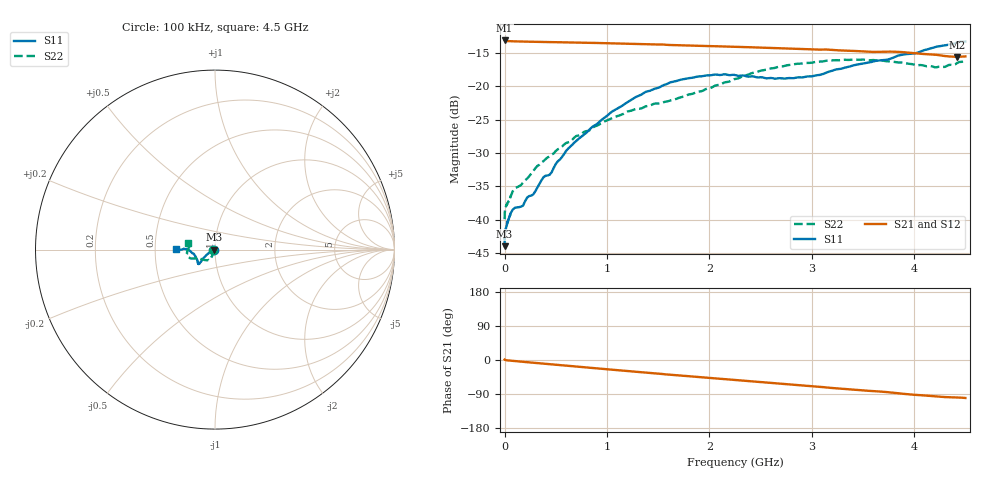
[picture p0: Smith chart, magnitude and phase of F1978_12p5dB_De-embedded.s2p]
! Integrated Device Technology
! Corporate Headquarters
! 6024 Silver Creek Valley Road
! San Jose, CA 95138  USA
! Phone:  1-408-284-8200
! Toll Free:  1-800-223-1366
! Webpage:  http://www.idt.com/
! Timing and RF Division
! 515 Groton Road, Suite 102
! Westford, MA 01886-6024
! Device:  F1978
! Description: 6-bit, 75 ohm, 0.5 dB Digital Step Attenuator
! Frequency:  5.0 MHz -  3.00 GHz
! Package:  4x4 mm QFN Plastic Package: 20 pin
! Ports:  2 RF, 11 DC
!  Pin  1  = D5 (16 dB)
!  Pin  2  = RF1  =  Port 1
!  Pin  3  = Serial Data In (DATA)
!  Pin  4  = Serial Clock (CLK)
!  Pin  5  = Serial Latch Enable (LE)
!  Pin  6  = VDD
!  Pin  7  = NC
!  Pin  8  = NC
!  Pin  9  = NC
!  Pin 10  = GND
!  Pin 11  = GND
!  Pin 12  = NC
!  Pin 13  = VMODE
!  Pin 14  = RF2  =  Port 2
!  Pin 15  = D4 (8 dB)
!  Pin 16  = D3 (4 dB)
!  Pin 17  = D2 (2 dB)
!  Pin 18  = NC
!  Pin 19  = D1 (1 dB)
!  Pin 20  = D0 (0.5 dB)
! State:  25
! Atten State:  12.5 dB
! Voltage:  +3.30 Volts
! Current:  0.561 mA
! Data:  The device was measured on a F1975 evaluation board which has
!  individual transmission lines to the RF pins.  Data was collected
!  using a calibrated network analyzer.  The evaluation board was
!  de-embedded using Automatic Fixture Removal (AFR).
!  The reference plane is the edge of the package pin.
! Misc:
!  Action Tracker AT0416
! Date Measured:  2018-02-08
! Date:  2018-03-26  MJV
! Note:
!  Integrated Device Technology supplies this data as a sample of measured
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# GHz S dB R 75
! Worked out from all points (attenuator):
!   291 points, 100 kHz to 4.5 GHz, reference 75 ohm
!   highest |S21| = -13.14 dB at 100 kHz (marker M1); lowest = -15.6 dB at 4.42 GHz (marker M2)
!   lowest |S11| = -44.0 dB at 100 kHz (marker M3), VSWR 1.01, Z = 74.1 - j0.013 ohm
!   |S11| at or under -10 dB: start of sweep to end of sweep
!   |S22| runs from -39.9 to -16.0 dB; largest |S21 - S12| = 0.00017
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0.0001  -43.96 -179.2  -13.14 1.2  -13.15 1.2  -39.93 -178.0
0.0005  -42.90 -175.7  -13.17 1.1  -13.17 1.1  -39.48 -177.0
0.002  -42.23 -174.5  -13.19 0.8  -13.19 0.8  -38.86 -175.4
0.014  -41.14 -172.1  -13.22 -0.6  -13.22 -0.6  -38.01 -171.0
0.08  -38.48 -163.3  -13.27 -2.3  -13.27 -2.3  -35.73 -156.9
0.18  -37.89 -159.1  -13.31 -4.8  -13.31 -4.8  -34.44 -136.9
0.22  -36.69 -159.0  -13.32 -5.8  -13.32 -5.8  -33.84 -132.0
0.32  -35.19 -159.4  -13.35 -8.2  -13.35 -8.2  -31.94 -124.8
0.38  -33.63 -155.9  -13.37 -9.6  -13.37 -9.6  -31.22 -120.6
0.46  -32.87 -156.9  -13.39 -11.5  -13.39 -11.5  -30.25 -117.9
0.6  -29.70 -154.5  -13.43 -14.9  -13.43 -14.9  -28.51 -114.7
0.76  -27.43 -149.7  -13.48 -18.7  -13.48 -18.7  -27.01 -114.3
1.06  -23.70 -145.5  -13.58 -25.8  -13.57 -25.8  -24.71 -116.2
1.52  -20.11 -139.5  -13.74 -36.4  -13.74 -36.4  -22.56 -127.7
1.88  -18.56 -138.0  -13.94 -44.6  -13.94 -44.6  -20.84 -142.7
2.26  -18.36 -141.4  -14.09 -53.1  -14.09 -53.1  -18.89 -154.4
2.64  -18.87 -152.5  -14.29 -61.6  -14.28 -61.6  -17.25 -158.8
3.02  -18.45 -167.6  -14.49 -69.7  -14.49 -69.7  -16.41 -163.1
3.76  -15.93 179.4  -14.82 -85.4  -14.82 -85.4  -16.29 -178.2
4.2  -14.15 -179.8  -15.28 -95.8  -15.28 -95.8  -17.16 169.9
4.42  -13.44 -179.5  -15.61 -99.0  -15.60 -99.0  -16.51 166.8
4.5  -13.30 178.6  -15.53 -100.2  -15.53 -100.2  -16.09 165.7
